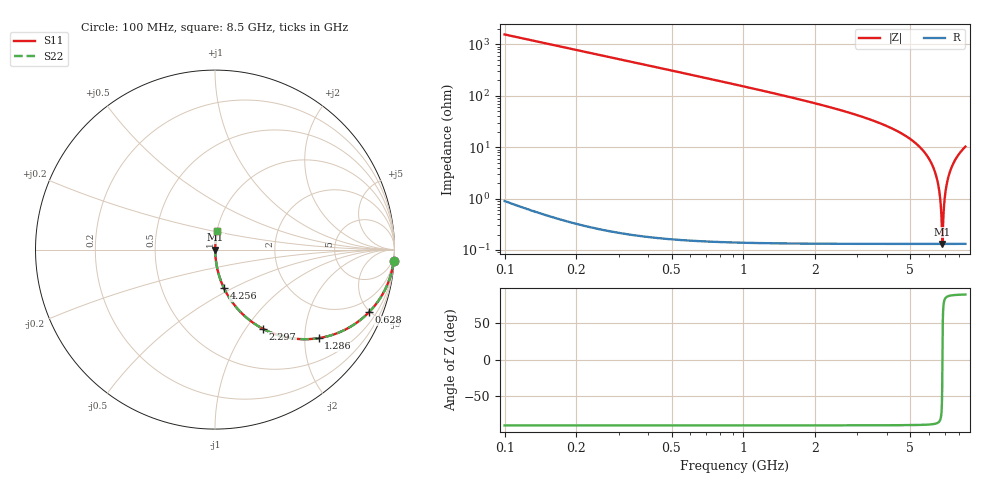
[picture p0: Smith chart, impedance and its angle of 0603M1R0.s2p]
! Created Wed Apr 18 12:05:54 2012
# hz S ma R 50
! 2 Port Network Data from SP1.SP block
! freq  magS11  angS11  magS21  angS21  magS12  angS12  magS22  angS22
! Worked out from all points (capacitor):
!   8401 points, 100 MHz to 8.5 GHz, reference 50 ohm
!   read as one part in series: C = 1.02 pF near 142 MHz
!   lowest |Z| = 131 mohm at 6.811 GHz (marker M1)
!   series resonance near 6.811 GHz, so ESL is about 540 pH
!   S11 on the Smith chart (normalised r, x): 100 MHz: 1, -31; 628 MHz: 1.00, -4.93; 1.286 GHz: 1.00, -2.34; 2.297 GHz: 1.00, -1.20; 4.256 GHz: 1.00, -0.45; 8.5 GHz: 1.00, +0.21
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1e8  0.9979 -3.7  0.06397 86.3  0.06397 86.3  0.9979 -3.7
3.06e8  0.9812 -11.1  0.1928 78.9  0.1928 78.9  0.9812 -11.1
6.28e8  0.9264 -22.1  0.376 67.9  0.376 67.9  0.9264 -22.1
1.286e9  0.7598 -40.5  0.6493 49.4  0.6493 49.4  0.7598 -40.5
1.5e9  0.703 -45.3  0.7102 44.7  0.7102 44.7  0.703 -45.3
2.297e9  0.5153 -58.9  0.8559 31.0  0.8559 31.0  0.5153 -58.9
2.9e9  0.4028 -66.1  0.9141 23.8  0.9141 23.8  0.4028 -66.1
4.256e9  0.2179 -77.1  0.9747 12.6  0.9747 12.6  0.2179 -77.1
4.3e9  0.2131 -77.4  0.9758 12.3  0.9758 12.3  0.2131 -77.4
5.7e9  0.08174 -84.4  0.9953 4.7  0.9953 4.7  0.08174 -84.4
6.188e9  0.044 -85.8  0.9977 2.5  0.9977 2.5  0.044 -85.8
6.506e9  0.02105 -85.2  0.9985 1.2  0.9985 1.2  0.02105 -85.2
6.68e9  0.009014 -81.1  0.9986 0.5  0.9986 0.5  0.009014 -81.1
6.732e9  0.005524 -75.9  0.9987 0.3  0.9987 0.3  0.005524 -75.9
6.787e9  0.002099 -51.2  0.9987 0.1  0.9987 0.1  0.002099 -51.2
6.811e9  0.001313 -0.9  0.9987 0.0  0.9987 0.0  0.001313 -0.9
6.836e9  0.002114 51.5  0.9987 -0.1  0.9987 -0.1  0.002114 51.5
6.889e9  0.005359 75.5  0.9987 -0.3  0.9987 -0.3  0.005359 75.5
6.939e9  0.00861 80.7  0.9987 -0.5  0.9987 -0.5  0.00861 80.7
7.1e9  0.01907 85.0  0.9985 -1.1  0.9985 -1.1  0.01907 85.0
7.605e9  0.05056 85.6  0.9974 -2.9  0.9974 -2.9  0.05056 85.6
8.5e9  0.1018 83.4  0.9935 -5.8  0.9935 -5.8  0.1018 83.4
